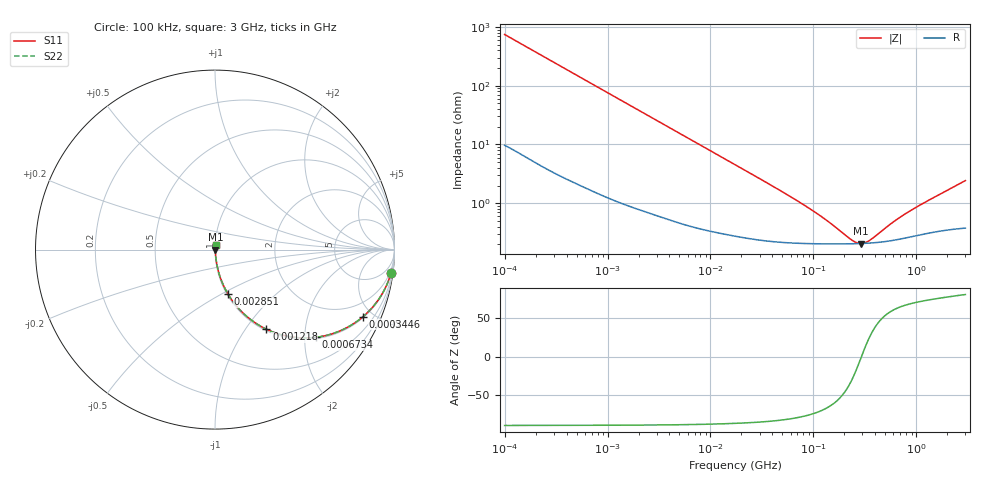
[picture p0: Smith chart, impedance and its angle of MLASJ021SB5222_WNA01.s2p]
! MLASJ021SB5222_WNA01  S-PARAMETER MODEL  ( Standard Model )
! Model Generated by TAIYO YUDEN Corporation (http://www.ty-top.com)
! Version 1.0
! TAIYO YUDEN Control No. 220901
! Copyright(c) 2022 TAIYO YUDEN CO.,LTD. All Rights Reserved.
! Product Description (link to TY-COMPAS)
! https://ds.yuden.co.jp/TYCOMPAS/or/detail?pn=MLASJ021SB5222KWNA01&u=M
! Products Name : Multilayer Ceramic Capacitors
! Characteristics :
!  Capacitance : 2200 [pF] , Rated Voltage : 6.3 [V] , TCC : X5R
!  Case Size : 0.25 x 0.125 / 0.0098 x 0.0049 [mm/inch] , Thickness : 0.125 / 0.0049 [mm/inch]
!  (Conditions: Temperature = 25 [degC] , DC Bias Voltage = 0 [V])
! External Node Assignments :
!  1  o---| |---o  2
! GND o---------o GND
! Frequency Range : 100kHz  -  3GHz  [ 401 STEP ]
# MHZ S RI R 50
! Freq[MHz].  S11 Real  S11 Imag  S21 Real  S21 Imag  S12 Real  S12 Imag  S22 Real  S22 Imag
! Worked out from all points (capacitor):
!   401 points, 100 kHz to 3 GHz, reference 50 ohm
!   read as one part in series: C = 2.12 nF near 105.3 kHz
!   lowest |Z| = 206 mohm at 287.5 MHz (marker M1)
!   series resonance near 292.7 MHz, so ESL is about 140 pH
!   S11 on the Smith chart (normalised r, x): 100 kHz: 1, -15; 344.6 kHz: 1.06, -4.40; 673.4 kHz: 1.03, -2.26; 1.218 MHz: 1.02, -1.26; 2.851 MHz: 1.01, -0.54; 3 GHz: 1.01, +0.05
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0.1  0.9809 -0.1306  0.0191 0.1306  0.0191 0.1306  0.9809 -0.1306
0.200542  0.9312 -0.2467  0.0688 0.2467  0.0688 0.2467  0.9312 -0.2467
0.344552  0.8252 -0.3732  0.1748 0.3732  0.1748 0.3732  0.8252 -0.3732
0.562235  0.6443 -0.4716  0.3557 0.4716  0.3557 0.4716  0.6443 -0.4716
0.673391  0.5601 -0.489  0.4399 0.489  0.4399 0.489  0.5601 -0.489
0.894104  0.4225 -0.4861  0.5775 0.4861  0.5775 0.4861  0.4225 -0.4861
1.218153  0.286 -0.4434  0.714 0.4434  0.714 0.4434  0.286 -0.4434
1.839868  0.1531 -0.3504  0.8469 0.3504  0.8469 0.3504  0.1531 -0.3504
2.851441  0.0732 -0.249  0.9268 0.249  0.9268 0.249  0.0732 -0.249
3.161081  0.0612 -0.2278  0.9388 0.2278  0.9388 0.2278  0.0612 -0.2278
6.848882  0.0165 -0.1113  0.9835 0.1113  0.9835 0.1113  0.0165 -0.1113
17.7727  0.00464 -0.0439  0.9954 0.0439  0.9954 0.0439  0.00464 -0.0439
49.82709  0.00238 -0.0155  0.9976 0.0155  0.9976 0.0155  0.00238 -0.0155
97.38194  0.00209 -0.00726  0.9979 0.00726  0.9979 0.00726  0.00209 -0.00726
139.694  0.00204 -0.0044  0.998 0.0044  0.998 0.0044  0.00204 -0.0044
233.9019  0.00203 -0.00123  0.998 0.00123  0.998 0.00123  0.00203 -0.00123
287.4592  0.00205 -9.85e-05  0.998 9.85e-05  0.998 9.85e-05  0.00205 -9.85e-05
318.6746  0.00207 0.000464  0.9979 -0.000464  0.9979 -0.000464  0.00207 0.000464
353.2796  0.00209 0.00103  0.9979 -0.00103  0.9979 -0.00103  0.00209 0.00103
547.5153  0.00228 0.0036  0.9977 -0.0036  0.9977 -0.0036  0.00228 0.0036
990.4458  0.00284 0.00795  0.9972 -0.00795  0.9972 -0.00795  0.00284 0.00795
3000  0.00431 0.0238  0.9957 -0.0238  0.9957 -0.0238  0.00431 0.0238
